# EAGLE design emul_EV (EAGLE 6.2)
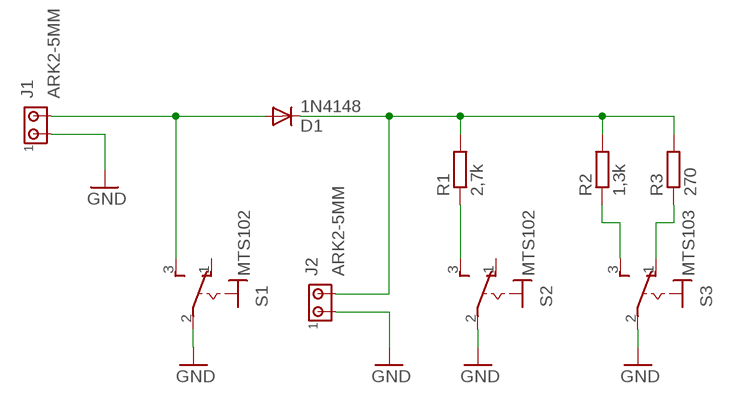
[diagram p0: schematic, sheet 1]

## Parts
D1  1N4148  1N4148DO35-7  [DO35-7]
J1  ARK2-5MM  [2PIN-5MM]
J2  ARK2-5MM  [2PIN-5MM]
R1  2,7k  R-EU_0207/7  [0207/7]
R2  1,3k  R-EU_0207/7  [0207/7]
R3  270  R-EU_0207/7  [0207/7]
S1  MTS102  PRZELACZNIK_MTS  [PRZELACZNIK_MTS_POJEDYNCZY]
S2  MTS102  PRZELACZNIK_MTS  [PRZELACZNIK_MTS_POJEDYNCZY]
S3  MTS103  PRZELACZNIK_MTS  [PRZELACZNIK_MTS_POJEDYNCZY]

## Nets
GND: J1.P$1 J2.P$1 S1.2(P) S2.2(P) S3.2(P)
N$1: D1.A J1.P$2 S1.3(S)
N$2: D1.C J2.P$2 R1.2 R2.2 R3.2
N$3: R1.1 S2.3(S)
N$4: R3.1 S3.1(O)
N$5: R2.1 S3.3(S)
Unconnected: S1.1(O) S2.1(O)

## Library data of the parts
D1 = diode:1N4148: DIODE
J1 J2 = zlacza_futrzak:ARK2: ARK 2
R1-R3 = rcl:R-EU_: RESISTOR, European symbol
S1-S3 = inne_futrzak:PRZELACZNIK_MTS: TOGGLE SWITCH Marquardt

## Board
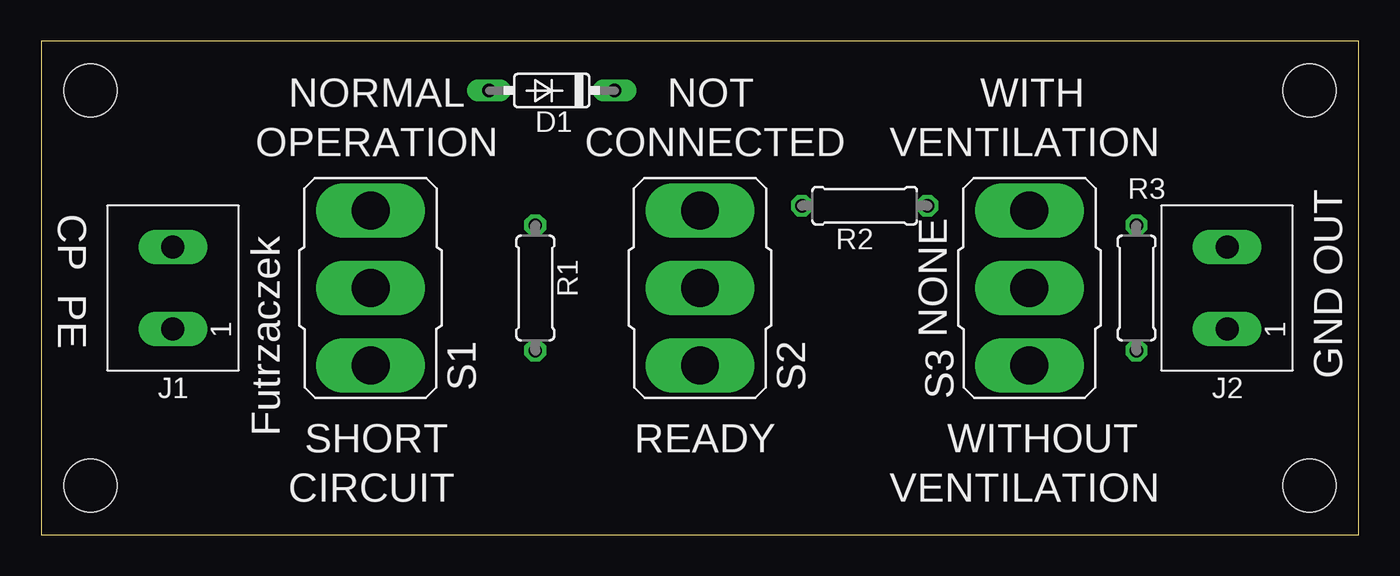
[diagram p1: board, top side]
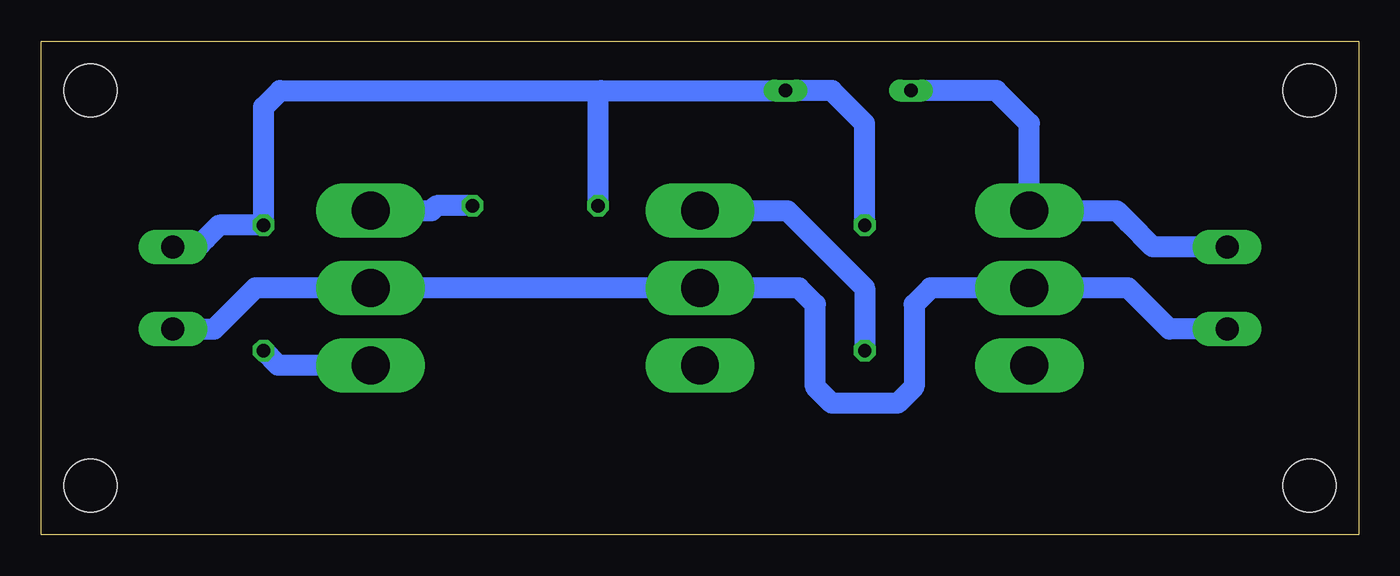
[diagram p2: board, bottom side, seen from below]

Size 80 x 30 mm. Coordinates in mm from the lower left corner, seen from the top.
Outline: 0,0 80,0 80,30 0,30 0,0
Copper layers (1*16): Top 0.035mm / dielectric 1.5mm / Bottom 0.035mm
Design rules: minimum track width 10mil, minimum drill 24mil, track to track 8mil, track to pad 8mil, pad to pad 8mil, via to via 8mil, smd to smd 8mil, copper to edge 40mil, drill to drill 8mil, minimum pad ring 10mil, minimum via ring 8mil, stop-mask expansion 4mil, vias tented up to drill 0mil, thermal gap 10mil
Holes 3.2 mm at 3,3 3,27 77,3 77,27

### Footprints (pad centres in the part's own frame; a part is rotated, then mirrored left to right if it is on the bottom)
DO35-7 = drill 0.813 long: A 3.81,0; C -3.81,0
2PIN-5MM = drill 1.4 long: P$1 -2.5,0; P$2 2.5,0
0207/7 = drill 0.813 octagon: 1 -3.81,0; 2 3.81,0
PRZELACZNIK_MTS_POJEDYNCZY = drill 2.3 long: 1 0,4.699; 2 0,0; 3 0,-4.699

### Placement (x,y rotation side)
D1  31,27 180 top
J1  8,15 90 top
J2  72,15 90 top
R1  30,15 90 top
R2  50,20 180 top
R3  66.5,15 90 top
S1  20,15 180 top
S2  40,15 180 top
S3  60,15 180 top

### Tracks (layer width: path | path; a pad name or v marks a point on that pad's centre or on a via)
GND
  Bottom 1.27: J1.P$1 11.5,12.5 14,15 S1.2 | S1.2 21,15 S1.2 | J2.P$1 69.5,12.5 69,13 67,15 S3.2 S2.2 34,15 33,14 33,9 32,8 28,8 27,9 27,14 26,15 S1.2
N$1
  Bottom 1.27: J1.P$2 12.5,17.5 14,19 14.7,19.7 S1.3 20,25 22,27 D1.A
N$2
  Bottom 1.27: R1.2 30,25 32,27 D1.C 46,27 | 46,27 65.5,27 66.5,26 R3.2 69.19,18.81 70,18 70.5,17.5 J2.P$2 | R2.2 46.19,26.81 46,27
N$3
  Bottom 1.27: S2.3 34.7,19.7 30,15 R1.1
N$4
  Bottom 1.27: S3.1 65.61,10.3 R3.1
N$5
  Bottom 1.27: R2.1 56,20 56.3,19.7 S3.3

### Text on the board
tPlace: NORMAL | NOT | WITH | OPERATION | CONNECTED | VENTILATION | CP PE | NONE | GND OUT | Futrzaczek | SHORT | READY | WITHOUT | CIRCUIT | VENTILATION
